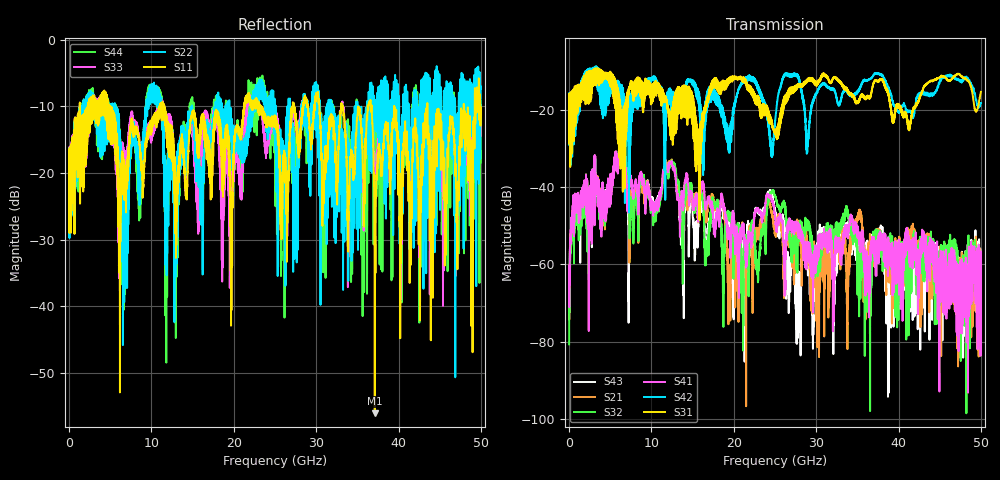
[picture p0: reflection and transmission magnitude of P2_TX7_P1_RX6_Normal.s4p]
!Keysight Technologies,N5225B,MY57041031,A.13.20.10
!Date: Friday, May 31, 2019 11:23:39
!Correction: S11(Full 4 Port(1,2,3,4))
!S12(Full 4 Port(1,2,3,4))
!S13(Full 4 Port(1,2,3,4))
!S14(Full 4 Port(1,2,3,4))
!S21(Full 4 Port(1,2,3,4))
!S22(Full 4 Port(1,2,3,4))
!S23(Full 4 Port(1,2,3,4))
!S24(Full 4 Port(1,2,3,4))
!S31(Full 4 Port(1,2,3,4))
!S32(Full 4 Port(1,2,3,4))
!S33(Full 4 Port(1,2,3,4))
!S34(Full 4 Port(1,2,3,4))
!S41(Full 4 Port(1,2,3,4))
!S42(Full 4 Port(1,2,3,4))
!S43(Full 4 Port(1,2,3,4))
!S44(Full 4 Port(1,2,3,4))
!S4P File: Measurements: <S11,S12,S13,S14>,
!<S21,S22,S23,S24>,
!<S31,S32,S33,S34>,
!<S41,S42,S43,S44>:
# Hz S  dB  R 50.0
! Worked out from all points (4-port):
!   5000 points, 10 MHz to 50 GHz, reference 50 ohm
!   strongest paths, dB at 10 MHz, 12.51 GHz, 25.01 GHz, 37.51 GHz, 50 GHz:
!     S31: -19.6, -21.1, -25.9, -12.8, -15.4
!     S42: -19.4, -15.6, -23.0, -10.9, -18.3
!     S41: -67.9, -33.9, -47.7, -55.4, -61.4
!     S32: -80.7, -33.5, -42.2, -52.9, -60.4
!     S21: -63.4, -33.4, -51.0, -52.1, -83.4
!     S43: -72.1, -33.6, -45.9, -55.6, -57.0
!   lowest |S11| = -56.0 dB at 37.12 GHz (marker M1), VSWR 1.00, Z = 49.8 - j0.0446 ohm
!   |S11| at or under -10 dB: 4.96 GHz to 11.03 GHz (6.066 GHz wide, 75.9 % of centre); 11.57 GHz to 21.26 GHz (9.683 GHz wide, 59 % of centre); 43.5 GHz to 47.91 GHz (4.409 GHz wide, 9.65 % of centre)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
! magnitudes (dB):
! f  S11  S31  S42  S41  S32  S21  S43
! 10 MHz  -20.2  -19.6  -19.4  -67.9  -80.7  -63.4  -72.1
! 6.25 GHz  -23.0  -22.0  -15.0  -29.3  -29.2  -29.4  -29.5
! 19.44 GHz  -17.7  -11.9  -31.1  -53.0  -46.9  -67.6  -49.8
! 24.15 GHz  -12.7  -22.2  -22.0  -42.1  -43.5  -43.2  -41.6
! 27.86 GHz  -15.2  -14.1  -11.5  -50.9  -51.5  -49.6  -65.5
! 37.12 GHz  -56.0  -12.6  -10.7  -55.3  -55.8  -55.9  -53.8
! 50 GHz  -11.1  -15.4  -18.3  -61.4  -60.4  -83.4  -57.0
